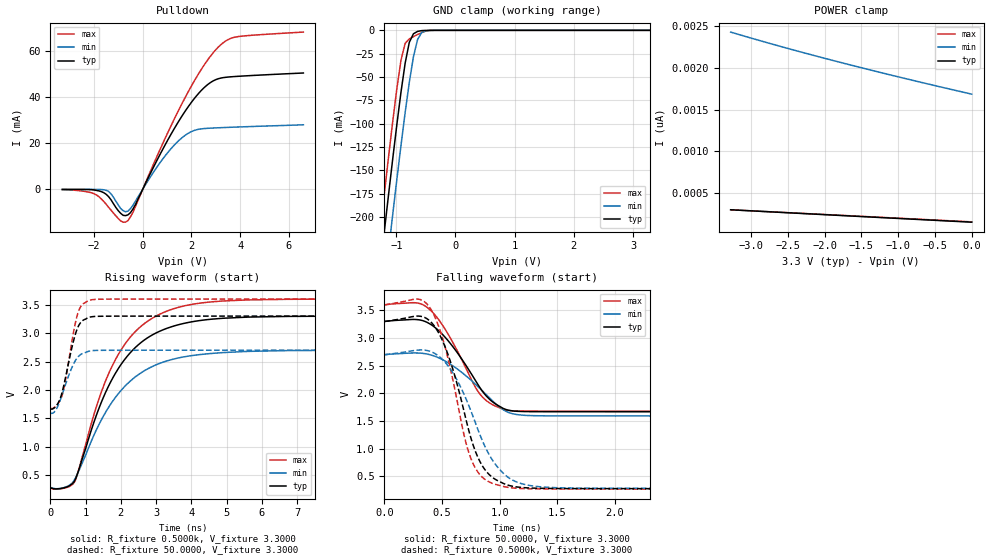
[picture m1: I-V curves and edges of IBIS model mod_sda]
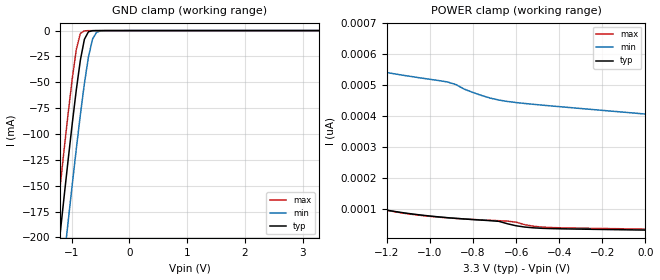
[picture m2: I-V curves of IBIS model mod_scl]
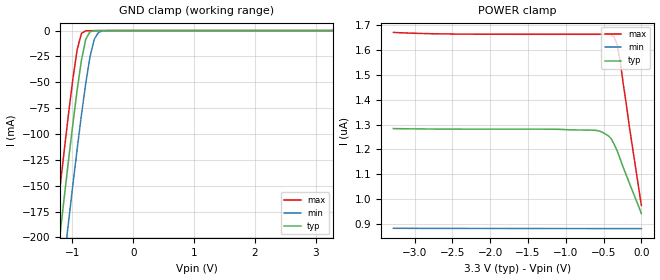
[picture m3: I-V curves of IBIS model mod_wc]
| IBIS (I/O, Buffer, Information, Specification) Model, officially
| electronic behavioral standard for Buffer structures of digital pins.
[IBIS ver]  4.0
[File name] m24c16_g2_tssop8.ibs
[File Rev]  1.0
[Date]   20 March 2015
[Source]   CAD & Design Services (Catania) - STMicroelectronics
[Notes]
   (Note1)  This IBIS model includes the TSSOP8 package data
   (Note2)  This IBIS model has some Notes about the non-monotonicity
   of the I-V curves, but they are not indicative of problems
   inside the model;
[Copyright] (c) 2015 STMicroelectronics
|   Component M24C16
[Component] M24C16
[Manufacturer] STMicroelectronics
[Package]
| variable   typ   min   max
R_pkg   0.0   0.0   0.0
L_pkg   0.0H   0.0H   0.0H
C_pkg   0.0F   0.0F   0.0F
[Pin]  signal_name   model_name   R_pin   L_pin   C_pin
1   NC   NC   NA   NA   NA
2   NC   NC   NA   NA   NA
3   NC   NC   NA   NA   NA
4   VSS   GND   NA   NA   NA
5   SDA   mod_sda   NA   NA   NA
6   SCL   mod_scl   NA   NA   NA
7   WCN   mod_wc   NA   NA   NA
8   VCC   POWER   NA   NA   NA
[Package Model]  182696_TSSOP8
[Define Package Model]  182696_TSSOP8
[Manufacturer]  STMicroelectronics
[OEM]  STMicroelectronics
[Description]  8 pin TSSOP package
[Number Of Pins]  8
[Pin Numbers]
|Pin Num   Terminal Name
1   | net1
2   | net2
3   | net3
4   | net4_GND
5   | net5
6   | net6
7   | net7
8   | net8_VDD
[Model Data]
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[End Model Data]
[End Package Model]
| Models and submodels in the file (3): mod_sda (I/O_open_drain), mod_scl (Input), mod_wc (Input)
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|   Model mod_sda
[Model]   mod_sda
Model_type I/O_open_drain
Polarity   Non-Inverting
Vinl   =   1.000V
Vinh   =   2.300V
Vmeas  =   1.650V
Cref   =   10pF
Rref   =   1k
Vref   =   3.300V
C_comp   2.668pF   2.547pF   2.925pF
[Temperature Range]  25.0000   0.1250k   -40.0000
[Voltage Range]   3.3000V   2.7000V   3.6000V
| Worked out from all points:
|   slope of the pulldown table from 0 to 0.495 V, typ, clamps not added: 46.4 ohm
|   GND clamp passes 1 mA (typ) near -0.63 V on its own axis
|   rising waveform, R_fixture 0.5000k, V_fixture 3.3000: 20-80 % time 1.37ns typ, 1.44ns min, 1.32ns max; typ from 0.277 V to 3.3 V
|   rising waveform, R_fixture 50.0000, V_fixture 3.3000: 20-80 % time 358ps typ, 400ps min, 326ps max; typ from 1.67 V to 3.3 V
|   falling waveform, R_fixture 50.0000, V_fixture 3.3000: 20-80 % time 323ps typ, 357ps min, 294ps max; typ from 3.3 V to 1.67 V
|   falling waveform, R_fixture 0.5000k, V_fixture 3.3000: 20-80 % time 251ps typ, 310ps min, 218ps max; typ from 3.3 V to 0.277 V
[Pulldown]
|Voltage   I(typ)   I(min)   I(max)
-3.3V     -30.12uA   -8.2uA     -108.8uA
-2.1V     -133.3uA   -10.15uA   -1.483mA
-1.5V     -2.122mA   -400.4uA   -6.415mA
-900mV    -10.41mA   -8.32mA    -13.69mA
-700mV    -11.37mA   -9.715mA   -14.18mA
-300mV    -6.676mA   -5.187mA   -7.487mA
700mV     14.87mA    11.37mA    16.95mA
1.5V      29.85mA    21.3mA     34.77mA
2.3V      41.61mA    26.03mA    50.15mA
3V        47.52mA    26.63mA    60.44mA
3.8V      48.9mA     26.98mA    65.96mA
6.6V      50.41mA    27.98mA    68.13mA
[GND_clamp]
|Voltage   I(typ)   I(min)   I(max)
-3.3V     -1.447A    -1.503A    -1.41A
-1.27V    -253.6mA   -313.5mA   -213.1mA
-1.2V     -214.3mA   -274.2mA   -173.7mA
-1.13V    -175.5mA   -235.3mA   -135.1mA
-1.06V    -137.5mA   -197mA     -97.61mA
-920mV    -65.95mA   -122.9mA   -31.83mA
-850mV    -35.13mA   -87.93mA   -13.93mA
-780mV    -12.87mA   -55.67mA   -9.13mA
-710mV    -3.674mA   -28.28mA   -6.723mA
-640mV    -1.164mA   -9.757mA   -4.512mA
-430mV    -26.5uA    -152.5uA   -68.17uA
3.28V     153.2pA    1.805nA    143.9pA
[POWER_clamp]
|Voltage   I(typ)   I(min)   I(max)
-3.28V    302.7pA    2.428nA    302.4pA
-2.6V     271.6pA    2.257nA    272.4pA
-1.8V     235.2pA    2.069nA    237.1pA
-960mV    197.2pA    1.885nA    200.2pA
0V        154.1pA    1.686nA    158pA
[Ramp]
| variable   typ   min   max
dV/dt_r  0.9793/0.3929n   0.6466/0.4875n   1.1532/0.3632n
dV/dt_f  0.9793/0.3633n   0.6466/0.4054n   1.1532/0.3175n
R_load = 50.0000
[Rising Waveform]
R_fixture= 0.5000k
V_fixture= 3.3000   | New Temp 105
V_fixture_min= 2.7000
V_fixture_max= 3.6000
|time   V(typ)   V(min)   V(max)
0s        277mV      283mV      269.8mV
380ps     275.1mV    279.1mV    269.1mV
670ps     379.4mV    399.9mV    362mV
1.34ns    1.609V     1.339V     1.767V
1.78ns    2.22V      1.811V     2.452V
2.34ns    2.703V     2.194V     2.981V
2.98ns    2.997V     2.437V     3.294V
3.78ns    3.17V      2.581V     3.477V
4.89ns    3.262V     2.657V     3.566V
10ns      3.3V       2.7V       3.6V
[Rising Waveform]
R_fixture= 50.0000
V_fixture= 3.3000   |  New Temp 105
V_fixture_min= 2.7000
V_fixture_max= 3.6000
|time   V(typ)   V(min)   V(max)
0s        1.668V     1.592V     1.678V
180ps     1.728V     1.672V     1.729V
340ps     1.969V     1.924V     1.913V
440ps     2.241V     2.108V     2.199V
640ps     2.817V     2.431V     2.95V
720ps     2.997V     2.525V     3.203V
800ps     3.126V     2.59V      3.383V
920ps     3.221V     2.643V     3.51V
1.12ns    3.282V     2.686V     3.58V
10ns      3.3V       2.7V       3.6V
[Falling Waveform]
R_fixture= 50.0000
V_fixture= 3.3000   | New Temp 105 (Min)
V_fixture_min= 2.7000
V_fixture_max= 3.6000
|time   V(typ)   V(min)   V(max)
0s        3.3V       2.7V       3.6V
260ps     3.336V     2.731V     3.639V
390ps     3.261V     2.702V     3.521V
470ps     3.135V     2.643V     3.333V
570ps     2.907V     2.53V      3.007V
830ps     2.099V     2.086V     1.983V
950ps     1.829V     1.84V      1.783V
1.09ns    1.69V      1.646V     1.689V
1.49ns    1.669V     1.594V     1.679V
10ns      1.668V     1.592V     1.678V
[Falling Waveform]
R_fixture= 0.5000k
V_fixture= 3.3000
V_fixture_min= 2.7000   | New 105 Temp
V_fixture_max= 3.6000
|time   V(typ)   V(min)   V(max)
0s        3.3V       2.7V       3.6V
290ps     3.397V     2.783V     3.704V
390ps     3.316V     2.764V     3.561V
550ps     2.711V     2.503V     2.642V
690ps     1.68V      1.985V     1.251V
770ps     1.063V     1.576V     725.4mV
890ps     574.4mV    964.5mV    421.3mV
1.07ns    343.8mV    488mV      302.7mV
1.69ns    280mV      288.7mV    272.4mV
10ns      277mV      283mV      269.8mV
|   Model mod_scl
[Model]   mod_scl
Model_type Input
Vinl   =   1.000V
Vinh   =   2.300V
C_comp   2.119pF   2.024pF   2.323pF
[Temperature Range]  25.0000   0.1250k   -40.0000
[Voltage Range]   3.3000V   2.7000V   3.6000V
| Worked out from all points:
|   GND clamp passes 1 mA (typ) near -0.70 V on its own axis
[GND_clamp]
|Voltage   I(typ)   I(min)   I(max)
-3.3V     -1.356A    -1.413A    -1.314A
-1.34V    -270.6mA   -330.9mA   -225.1mA
-1.27V    -233.3mA   -293.7mA   -187.7mA
-1.2V     -196.3mA   -256.7mA   -150.7mA
-1.13V    -159.9mA   -220.1mA   -114.5mA
-1.06V    -124.2mA   -184mA     -79.36mA
-920mV    -57.24mA   -114.3mA   -18.31mA
-850mV    -28.61mA   -81.46mA   -2.742mA
-780mV    -8.435mA   -51.17mA   -243.2uA
-640mV    -136.1uA   -8.386mA   -70.24uA
-500mV    -14.94uA   -269.3uA   -31.6uA
3.28V     1.285uA    880.8nA    1.664uA
[POWER_clamp]
|Voltage   I(typ)   I(min)   I(max)
-3.28V    711.2nA    9.987nA    1.809uA
-2.12V    697.2pA    804.4pA    1.271nA
-1.96V    450.4pA    719.2pA    707.2pA
-1.84V    330.7pA    672pA      466.1pA
-1.72V    247.9pA    635.1pA    315.9pA
-1.6V     190.4pA    605.7pA    222pA
-1.44V    139.9pA    575pA      148.9pA
-1.28V    108.5pA    551.2pA    109.2pA
-1.04V    81.47pA    523.3pA    80.3pA
-640mV    53.44pA    447.8pA    62.09pA
-480mV    38.86pA    436pA      42.8pA
0V        33.08pA    407.2pA    36.22pA
|   Model mod_wc
[Model]   mod_wc
Model_type Input
Vinl   =   1.000V
Vinh   =   2.300V
C_comp   2.119pF   2.024pF   2.323pF
[Temperature Range]  25.0000   0.1250k   -40.0000
[Voltage Range]   3.3000V   2.7000V   3.6000V
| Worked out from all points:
|   GND clamp passes 1 mA (typ) near -0.70 V on its own axis
[GND_clamp]
|Voltage   I(typ)   I(min)   I(max)
-3.3V     -1.356A    -1.413A    -1.314A
-1.34V    -270.6mA   -330.9mA   -225.1mA
-1.27V    -233.3mA   -293.7mA   -187.7mA
-1.2V     -196.3mA   -256.7mA   -150.7mA
-1.13V    -159.9mA   -220.1mA   -114.5mA
-1.06V    -124.2mA   -184mA     -79.36mA
-920mV    -57.24mA   -114.3mA   -18.31mA
-850mV    -28.61mA   -81.46mA   -2.742mA
-780mV    -8.435mA   -51.17mA   -243.2uA
-640mV    -136.1uA   -8.386mA   -70.24uA
-500mV    -14.94uA   -269.3uA   -31.6uA
3.28V     1.285uA    880.8nA    1.664uA
[POWER_clamp]
|Voltage   I(typ)   I(min)   I(max)
-3.28V    1.284uA    882nA      1.672uA
-2.48V    1.282uA    881.5nA    1.665uA
-640mV    1.277uA    880.8nA    1.664uA
-520mV    1.27uA     880.8nA    1.664uA
-440mV    1.256uA    880.7nA    1.664uA
-400mV    1.244uA    880.7nA    1.663uA
-360mV    1.221uA    880.7nA    1.653uA
-320mV    1.194uA    880.7nA    1.621uA
-280mV    1.161uA    880.7nA    1.555uA
-240mV    1.128uA    880.7nA    1.465uA
-160mV    1.065uA    880.6nA    1.295uA
0V        941.6nA    880.5nA    974.1nA
